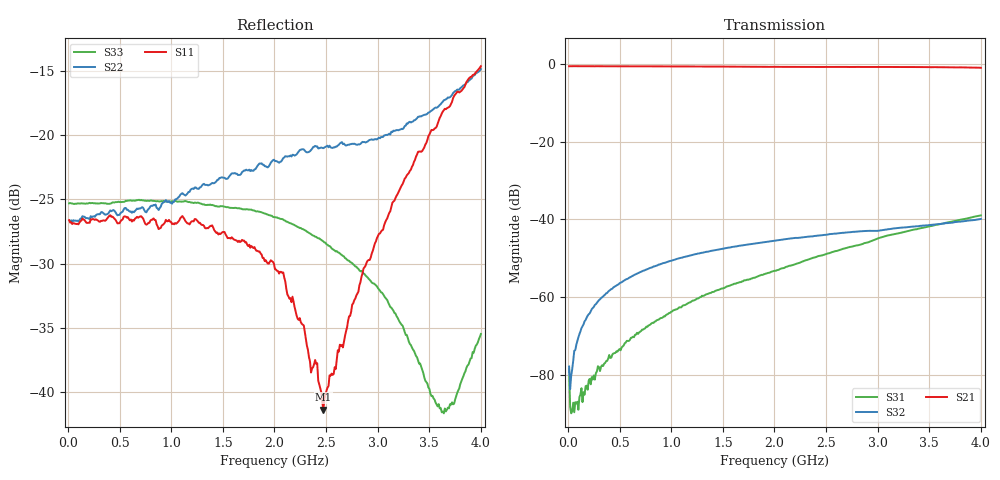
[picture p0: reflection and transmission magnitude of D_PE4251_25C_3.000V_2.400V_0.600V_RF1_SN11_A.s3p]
! Device ID: PE4251_SoldCshunt_081809
! Dir: c:\Test Bench Repositories\Bench_Software_CVI_Version_8\trunk\PSC 4Port_VNA Bench\datalog\4250\TEST\PE4251_SoldCshunt_081809\25C\3p000000\RF1
! Serial: 11
! Insertion: A
! Temp: 25C
! VDD: 3.000
! Control_Hi: 80.000
! Control_Lo: 20.000
! Logic State: RF1
! Port 1: RFC
! Port 2: RF1
! Port 3: RF2
! V1 = 0.60
! V2 = 2.40
! V3 = 0.60
! IDD: 5.140250e-05
! FILE NAME
! DATE 08/18/09  20:12
! CORRECTED  DATA
#  Hz  S  RI  R  50.00
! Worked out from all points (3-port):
!   401 points, 10 MHz to 4 GHz, reference 50 ohm
!   strongest paths, dB at 10 MHz, 1.008 GHz, 2.005 GHz, 3.002 GHz, 4 GHz:
!     S21: -0.6, -0.6, -0.7, -0.7, -1.0
!     S32: -77.9, -50.6, -45.4, -42.9, -39.9
!     S31: -78.6, -63.7, -53.2, -44.9, -39.0
!   lowest |S11| = -41.4 dB at 2.474 GHz (marker M1), VSWR 1.02, Z = 49.9 - j0.853 ohm
!   |S11| at or under -10 dB: start of sweep to end of sweep
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1e7  0.0466 -0.000268  0.9367 -0.00259  2.17e-05 1.67e-05
     0.9377 -0.00322  0.0465 -0.000153  6.16e-05 3.21e-05
     6.84e-05 -9.53e-05  4.96e-05 0.000118  0.0542 -0.000422
1.0975e8  0.0456 0.000234  0.9378 -0.0377  1.65e-05 -4.91e-05
          0.9377 -0.0379  0.0466 0.000192  3.73e-05 0.000334
          1.76e-05 -4.87e-05  3.47e-05 0.000332  0.0541 -0.00101
1.8955e8  0.0455 -0.000315  0.9358 -0.0644  5.28e-06 -8.49e-05
          0.9355 -0.0644  0.0474 -0.000724  5.53e-05 0.000572
          -4.59e-06 -6.41e-05  3.82e-05 0.000575  0.0541 -0.00136
4.98775e8  0.0452 -0.00378  0.9205 -0.1656  -0.00015 -0.000167
           0.9206 -0.1649  0.0488 -0.00304  0.000159 0.00149
           -0.000136 -0.000167  0.00016 0.0015  0.0546 -0.00451
1.017475e9  0.0425 -0.0154  0.8736 -0.3276  -0.000614 -0.000244
            0.873 -0.3271  0.0528 -0.0151  0.000486 0.00295
            -0.000622 -0.000256  0.000487 0.00295  0.0548 -0.00646
2.005e9  0.0268 -0.0135  0.7141 -0.5822  -0.00219 -0.000135
         0.714 -0.5822  0.0686 -0.0393  0.00112 0.0052
         -0.00219 -0.000132  0.00112 0.00522  0.0477 -0.00488
2.473825e9  -0.000501 -0.00854  0.6185 -0.6783  -0.00348 -0.000121
            0.6169 -0.6771  0.0628 -0.0627  0.00125 0.00615
            -0.00348 -0.000134  0.00125 0.00618  0.0385 -0.000961
2.8828e9  -0.0216 -0.0223  0.5222 -0.7552  -0.00498 0.000108
          0.5246 -0.7537  0.0408 -0.084  0.0013 0.00695
          -0.00498 0.0001  0.00133 0.00697  0.0283 0.00175
3.62095e9  -0.1015 -0.0661  0.3083 -0.8554  -0.00861 0.00183
           0.3094 -0.8561  -0.0485 -0.1241  0.000408 0.00876
           -0.00861 0.0018  0.000392 0.00877  0.00204 0.0081
4e9  -0.1666 -0.0804  0.1749 -0.8809  -0.0108 0.00324
     0.174 -0.878  -0.1282 -0.1267  -0.00026 0.0101
     -0.0108 0.00323  -0.00028 0.0101  -0.0139 0.00955
